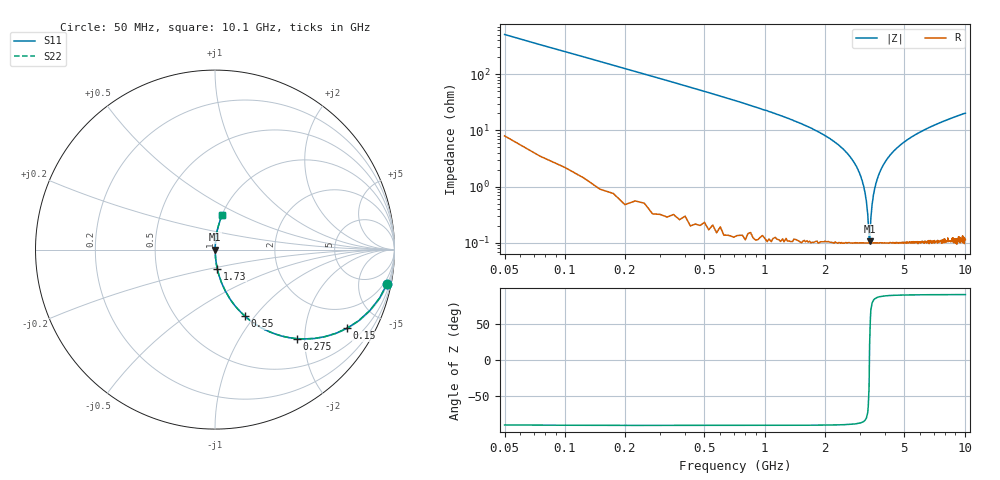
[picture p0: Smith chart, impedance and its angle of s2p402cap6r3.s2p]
! AVX Thin Film Operation		Date: April 2003
! Description: Accu-P® Series, Thin Film, SMD, RF Capacitor
! Part Number: 04025J6R3BBS
! 50 MHz  -  10.05 GHz
! Serial Measurements
# hz S db R 50
!	S11		S21		S12		S22
!	dB	Phase	dB	Phase	dB	Phase	dB	Phase
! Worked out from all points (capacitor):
!   400 points, 50 MHz to 10.1 GHz, reference 50 ohm
!   read as one part in series: C = 6.3 pF near 100 MHz
!   lowest |Z| = 106 mohm at 3.35 GHz (marker M1)
!   series resonance near 3.344 GHz, so ESL is about 360 pH
!   S11 on the Smith chart (normalised r, x): 50 MHz: 1, -10; 150 MHz: 1.02, -3.36; 275 MHz: 1.01, -1.83; 550 MHz: 1.00, -0.89; 1.73 GHz: 1.00, -0.22; 10.1 GHz: 1.00, +0.40
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5e7  -0.20 -11.2  -14.30 77.9  -14.30 77.9  -0.20 -11.2
1e8  -0.66 -21.5  -8.70 68.0  -8.70 68.0  -0.66 -21.5
1.5e8  -1.34 -30.7  -5.85 59.0  -5.85 59.0  -1.34 -30.7
2.75e8  -3.44 -47.5  -2.65 42.3  -2.65 42.3  -3.44 -47.5
5.5e8  -7.80 -65.7  -0.80 24.0  -0.80 24.0  -7.80 -65.7
1.73e9  -19.40 -83.3  -0.06 6.1  -0.06 6.1  -19.40 -83.3
2.48e9  -26.70 -86.1  -0.02 2.6  -0.02 2.6  -26.70 -86.1
2.98e9  -35.10 -85.7  -0.01 1.0  -0.01 1.0  -35.10 -85.7
3.13e9  -39.80 -83.8  -0.01 0.6  -0.01 0.6  -39.80 -83.8
3.23e9  -45.20 -79.2  -0.01 0.3  -0.01 0.3  -45.20 -79.2
3.28e9  -49.90 -71.7  -0.01 0.2  -0.01 0.2  -49.90 -71.7
3.33e9  -58.00 -37.5  -0.01 0.0  -0.01 0.0  -58.00 -37.5
3.35e9  -59.50 20.0  -0.01 -0.0  -0.01 -0.0  -59.50 20.0
3.4e9  -51.10 68.8  -0.01 -0.1  -0.01 -0.1  -51.10 68.8
3.45e9  -46.20 78.0  -0.01 -0.3  -0.01 -0.3  -46.20 78.0
3.55e9  -40.70 83.2  -0.01 -0.5  -0.01 -0.5  -40.70 83.2
3.8e9  -34.20 85.9  -0.01 -1.1  -0.01 -1.1  -34.20 85.9
4.25e9  -28.70 86.3  -0.01 -2.1  -0.01 -2.1  -28.70 86.3
5.08e9  -23.80 85.4  -0.03 -3.7  -0.03 -3.7  -23.80 85.4
6.75e9  -18.80 82.9  -0.07 -6.6  -0.07 -6.6  -18.80 82.9
8.43e9  -16.00 80.5  -0.12 -9.1  -0.12 -9.1  -16.00 80.5
1.01e10  -14.10 78.3  -0.18 -11.4  -0.18 -11.4  -14.10 78.3
